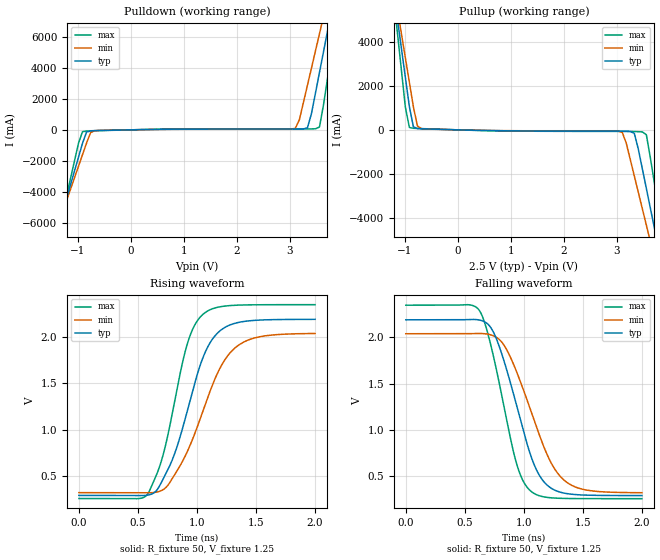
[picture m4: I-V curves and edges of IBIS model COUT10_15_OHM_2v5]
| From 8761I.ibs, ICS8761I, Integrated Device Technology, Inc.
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[Model] COUT10_15_OHM_2v5
Model_type   Output
Polarity   Non-Inverting
|   typ   min   max
C_comp   2pF   1.5pF   2.5pF
Vmeas = 1.25V
Rref = 50
Cref = 0
Vref = 1.25V
|   typ   min   max
[Voltage range]   2.5V   2.375V   2.625V
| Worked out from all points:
|   slope of the pulldown table from 0 to 0.375 V, typ, clamps not added: 15.7 ohm
|   slope of the pullup table from 0 to 0.375 V, typ, clamps not added: 16.9 ohm
|   rising waveform, R_fixture 50, V_fixture 1.25: 20-80 % time 271ps typ, 328ps min, 218ps max; typ from 0.289 V to 2.19 V
|   falling waveform, R_fixture 50, V_fixture 1.25: 20-80 % time 257ps typ, 305ps min, 212ps max; typ from 2.19 V to 0.289 V
[Pulldown]
|Voltage   I (typ)   I (min)   I (max)
-2.5V     -19.68A    -17.28A    -23.73A
-1.439V   -7.139A    -6.83A     -7.73A
-1.364V   -6.243A    -6.083A    -6.586A
-909.1mV  -868mA     -1.604A    -120mA
-833.3mV  -148.1mA   -858.1mA   -77.34mA
-681.8mV  -50.66mA   -56.35mA   -57.61mA
3.106V    52.05mA    102mA      60.73mA
3.333V    133.3mA    2.872A     61.18mA
3.561V    3.704A     6.201A     183.5mA
3.712V    6.369A     8.421A     3.314A
3.864V    9.036A     10.64A     6.72A
5V        29.06A     27.33A     32.31A
[Pullup]
|Voltage   I (typ)   I (min)   I (max)
-2.5V     29.11A     25.53A     35.17A
-1.136V   5.055A     5.495A     4.444A
-909.1mV  1.05A      2.158A     108.2mA
-833.3mV  137.8mA    1.047A     70.3mA
-681.8mV  48.38mA    53.62mA    56.56mA
3.106V    -62.59mA   -118.3mA   -71.54mA
3.333V    -157.8mA   -2.094A    -77.62mA
3.485V    -1.769A    -3.583A    -93.66mA
3.561V    -2.662A    -4.328A    -221.8mA
3.712V    -4.451A    -5.818A    -2.414A
3.864V    -6.24A     -7.309A    -4.698A
5V        -19.66A    -18.5A     -21.84A
[Ramp]
|   typ   min   max
dV/dt_r   1.522/0.426n   1.376/0.508n   1.676/0.344n
dV/dt_f   1.524/0.384n   1.378/0.458n   1.679/0.314n
R_load =   50.0000
[Rising Waveform]
R_fixture = 50
V_fixture = 1.25   |Vcc_typ
V_fixture_min = 1.1875 |Vcc_min
V_fixture_max = 1.3125 |Vcc_max
C_fixture = 0.0p
| Time   typ   min   max
0s        288.7mV    318.6mV    255.3mV
584.6ps   292.1mV    317.4mV    308.2mV
696.7ps   424.5mV    339.9mV    652.6mV
790.8ps   672.5mV    470.8mV    1.172V
922.9ps   1.225V     775.3mV    1.945V
1.057ns   1.797V     1.223V     2.251V
1.205ns   2.076V     1.688V     2.328V
1.357ns   2.158V     1.915V     2.344V
1.574ns   2.184V     2.011V     2.348V
2ns       2.19V      2.038V     2.349V
[Falling Waveform]
R_fixture = 50
V_fixture = 1.25   |Vcc_typ
V_fixture_min = 1.1875 |Vcc_min
V_fixture_max = 1.3125 |Vcc_max
C_fixture = 0.0p
| Time   typ   min   max
0s        2.19V      2.04V      2.349V
532.5ps   2.193V     2.04V      2.353V
624.6ps   2.188V     2.043V     2.289V
688.7ps   2.151V     2.037V     2.071V
778.8ps   1.948V     1.991V     1.585V
936.9ps   1.272V     1.633V     640.5mV
1.061ns   712mV      1.2V       334.7mV
1.183ns   419.5mV    773.5mV    271.8mV
1.363ns   310.3mV    432.8mV    257.5mV
2ns       288.9mV    319.9mV    255.3mV
